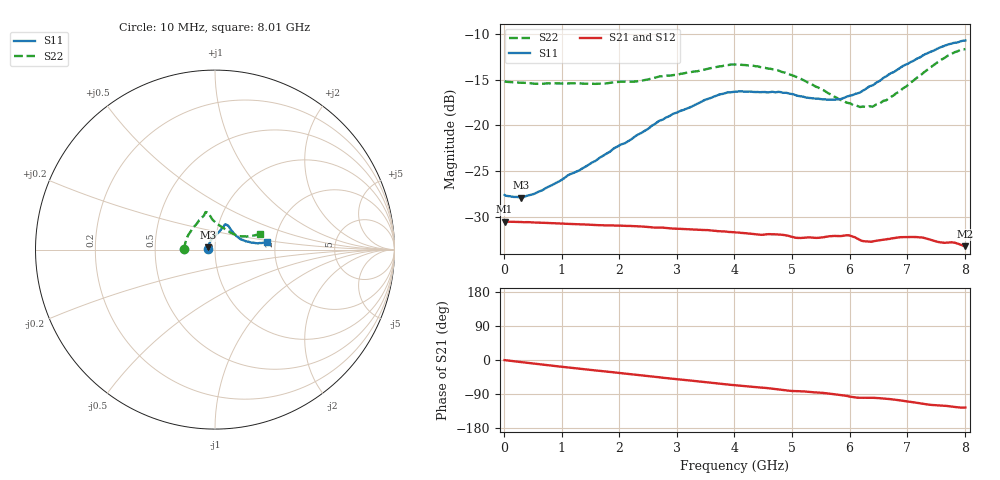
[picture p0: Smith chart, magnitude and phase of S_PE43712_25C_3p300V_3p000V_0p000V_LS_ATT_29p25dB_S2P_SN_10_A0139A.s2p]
! DEVICE ID: PE43712
! File Path: z:\PE43713\PE43713_CHAR_NOM_04292014\AMB\3p300\LS_ATT_29p25dB\PE43713_AMB_3p300V_3p000V_0p000V_LS_ATT_29p25dB_S2P_SN_10_A0139A.s2p
! Serial: 10
! Lot: A0139A
! Temp: 25C
! VDD: 3.300
! VSS: 0.000
! Control_Hi: 3.000
! Control_Lo: 0.000
! Attenuation Step: 29.25dB
! Port 1: RF1
! Port 2: RF2
! ThroughPath:1-2
! IDD: 0.0001459983
! ISS: -1.171e-007
#  Hz  S  RI  R  50
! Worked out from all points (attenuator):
!   801 points, 10 MHz to 8.01 GHz, reference 50 ohm
!   highest |S21| = -30.52 dB at 10 MHz (marker M1); lowest = -33.2 dB at 8.01 GHz (marker M2)
!   lowest |S11| = -27.9 dB at 290 MHz (marker M3), VSWR 1.08, Z = 46.3 + j1.23 ohm
!   |S11| at or under -10 dB: start of sweep to end of sweep
!   |S22| runs from -18.0 to -11.6 dB; largest |S21 - S12| = 0.00011
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1e7  -0.0416 0.000909  0.0298 -0.000147  0.0298 -0.00012  -0.1742 0.00127
2.9e8  -0.0381 0.0133  0.0295 -0.00279  0.0295 -0.00279  -0.1701 0.0197
6.5e8  -0.0337 0.0281  0.0287 -0.006  0.0287 -0.00599  -0.1637 0.0423
1.35e9  -0.021 0.054  0.0263 -0.0115  0.0263 -0.0115  -0.1476 0.0835
2.28e9  0.00951 0.0869  0.0219 -0.0177  0.0219 -0.0176  -0.1093 0.1354
2.68e9  0.025 0.1023  0.0194 -0.0196  0.0194 -0.0196  -0.0889 0.1624
3.5e9  0.0484 0.1297  0.014 -0.0228  0.014 -0.0228  -0.0594 0.1938
3.74e9  0.0533 0.1379  0.0122 -0.0234  0.0122 -0.0234  -0.0552 0.2032
4.01e9  0.0582 0.1415  0.0103 -0.0239  0.0103 -0.0239  -0.0522 0.2093
4.31e9  0.0617 0.1396  0.00827 -0.0241  0.00828 -0.0241  -0.0443 0.2079
4.75e9  0.072 0.1345  0.00546 -0.0247  0.00548 -0.0247  -0.0325 0.1978
5.08e9  0.0816 0.1207  0.00331 -0.024  0.00331 -0.024  -0.023 0.1826
5.35e9  0.0911 0.1073  0.00213 -0.0243  0.00208 -0.0242  -0.0139 0.167
5.81e9  0.1136 0.0799  -0.000835 -0.0248  -0.000783 -0.0248  0.0197 0.1381
5.98e9  0.1263 0.0709  -0.00252 -0.0249  -0.00249 -0.0249  0.0358 0.1278
6.17e9  0.1386 0.0602  -0.00399 -0.0234  -0.00392 -0.0234  0.0556 0.1135
6.4e9  0.1574 0.0521  -0.00395 -0.0228  -0.00386 -0.0228  0.0818 0.097
6.68e9  0.1852 0.0435  -0.00537 -0.0233  -0.00531 -0.0233  0.115 0.0817
7.15e9  0.2272 0.036  -0.00939 -0.0226  -0.00939 -0.0226  0.165 0.0733
7.56e9  0.2637 0.0375  -0.0116 -0.0199  -0.0116 -0.0198  0.2116 0.0783
7.81e9  0.2801 0.0406  -0.0126 -0.0191  -0.0126 -0.0191  0.2361 0.084
8.01e9  0.2886 0.0433  -0.0127 -0.0178  -0.0127 -0.0178  0.248 0.0848
